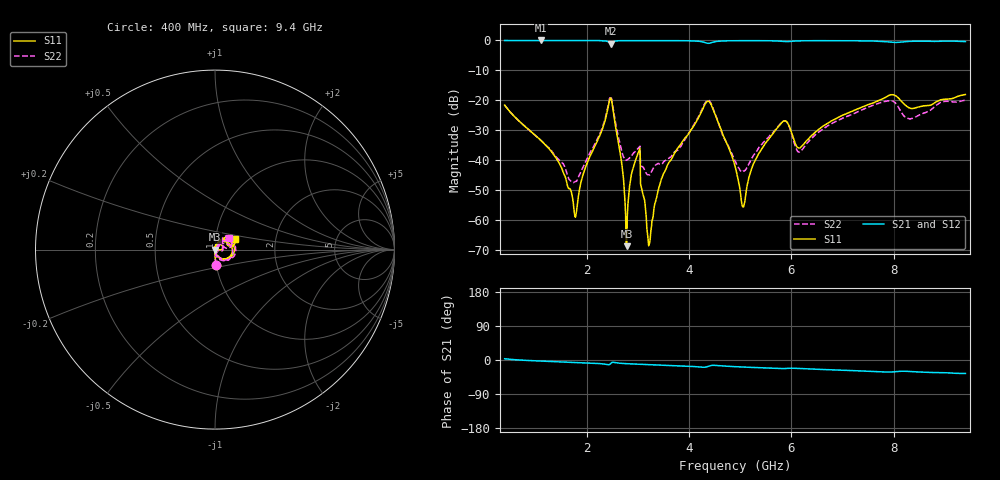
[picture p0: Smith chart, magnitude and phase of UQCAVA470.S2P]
!  Part Number  UQCAVA470	Mounting Orientation: Horizontal
!  Description: RF capacitors
!  Application: Coupling, Bypass, Tuning, DC Block
!  Filters, Matching
# GHZ S DB R 50
! Freq  |S11|  S11 Ph  |S21|  S21 Ph  |S12|  S12 Ph  |S22|  S22 Ph
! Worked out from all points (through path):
!   801 points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, 400 MHz to 9.4 GHz, reference 50 ohm
!   highest |S21| = -0.02 dB at 1.109 GHz (marker M1); lowest = -1.1 dB at 2.47 GHz (marker M2)
!   group delay of S21, straight-line fit = 11 ps
!   lowest |S11| = -68.6 dB at 2.785 GHz (marker M3), VSWR 1.00, Z = 50 + j0.033 ohm
!   |S11| at or under -10 dB: start of sweep to end of sweep
!   |S22| runs from -47.4 to -18.6 dB; largest |S21 - S12| = 0.0035
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0.4  -21.55 -86.0  -0.04 3.3  -0.06 3.3  -21.58 -86.0
1.109  -33.36 -92.5  -0.02 -2.9  -0.03 -2.8  -33.29 -87.4
1.491  -41.83 -98.3  -0.03 -5.0  -0.04 -4.9  -40.22 -72.3
1.773  -58.67 -168.7  -0.04 -6.4  -0.05 -6.4  -47.12 -6.4
1.908  -46.25 96.5  -0.04 -7.1  -0.05 -7.1  -43.07 34.3
2.47  -19.19 0.4  -1.07 -9.6  -1.08 -9.6  -18.60 -4.8
2.673  -39.18 -85.1  -0.10 -8.8  -0.11 -8.7  -35.87 -53.7
2.785  -68.56 117.9  -0.08 -9.8  -0.09 -9.7  -39.87 -7.5
2.886  -43.92 98.0  -0.07 -10.4  -0.09 -10.3  -38.24 21.4
2.999  -38.01 101.3  -0.07 -11.0  -0.08 -10.9  -36.15 36.8
3.213  -68.42 -140.9  -0.07 -12.2  -0.08 -12.1  -44.74 -14.9
3.404  -49.61 106.9  -0.07 -13.1  -0.08 -13.0  -41.02 10.7
4.36  -20.31 2.3  -0.95 -17.6  -0.95 -17.5  -19.93 -8.9
4.9  -41.84 -83.7  -0.10 -17.6  -0.11 -17.5  -40.11 -57.7
5.058  -55.48 -9.1  -0.10 -18.6  -0.10 -18.5  -43.56 -7.1
5.294  -39.96 65.2  -0.10 -19.9  -0.10 -19.8  -37.52 37.9
5.811  -27.42 39.4  -0.29 -22.8  -0.29 -22.7  -27.35 23.2
6.149  -35.89 23.4  -0.16 -22.4  -0.16 -22.3  -37.22 11.0
6.408  -31.53 57.5  -0.11 -23.9  -0.10 -23.8  -32.42 50.8
7.904  -18.35 36.4  -0.51 -31.8  -0.50 -31.7  -20.13 27.5
8.32  -22.60 20.5  -0.31 -30.4  -0.29 -30.2  -26.14 29.8
9.4  -18.03 28.0  -0.40 -35.5  -0.38 -35.4  -19.95 39.3
